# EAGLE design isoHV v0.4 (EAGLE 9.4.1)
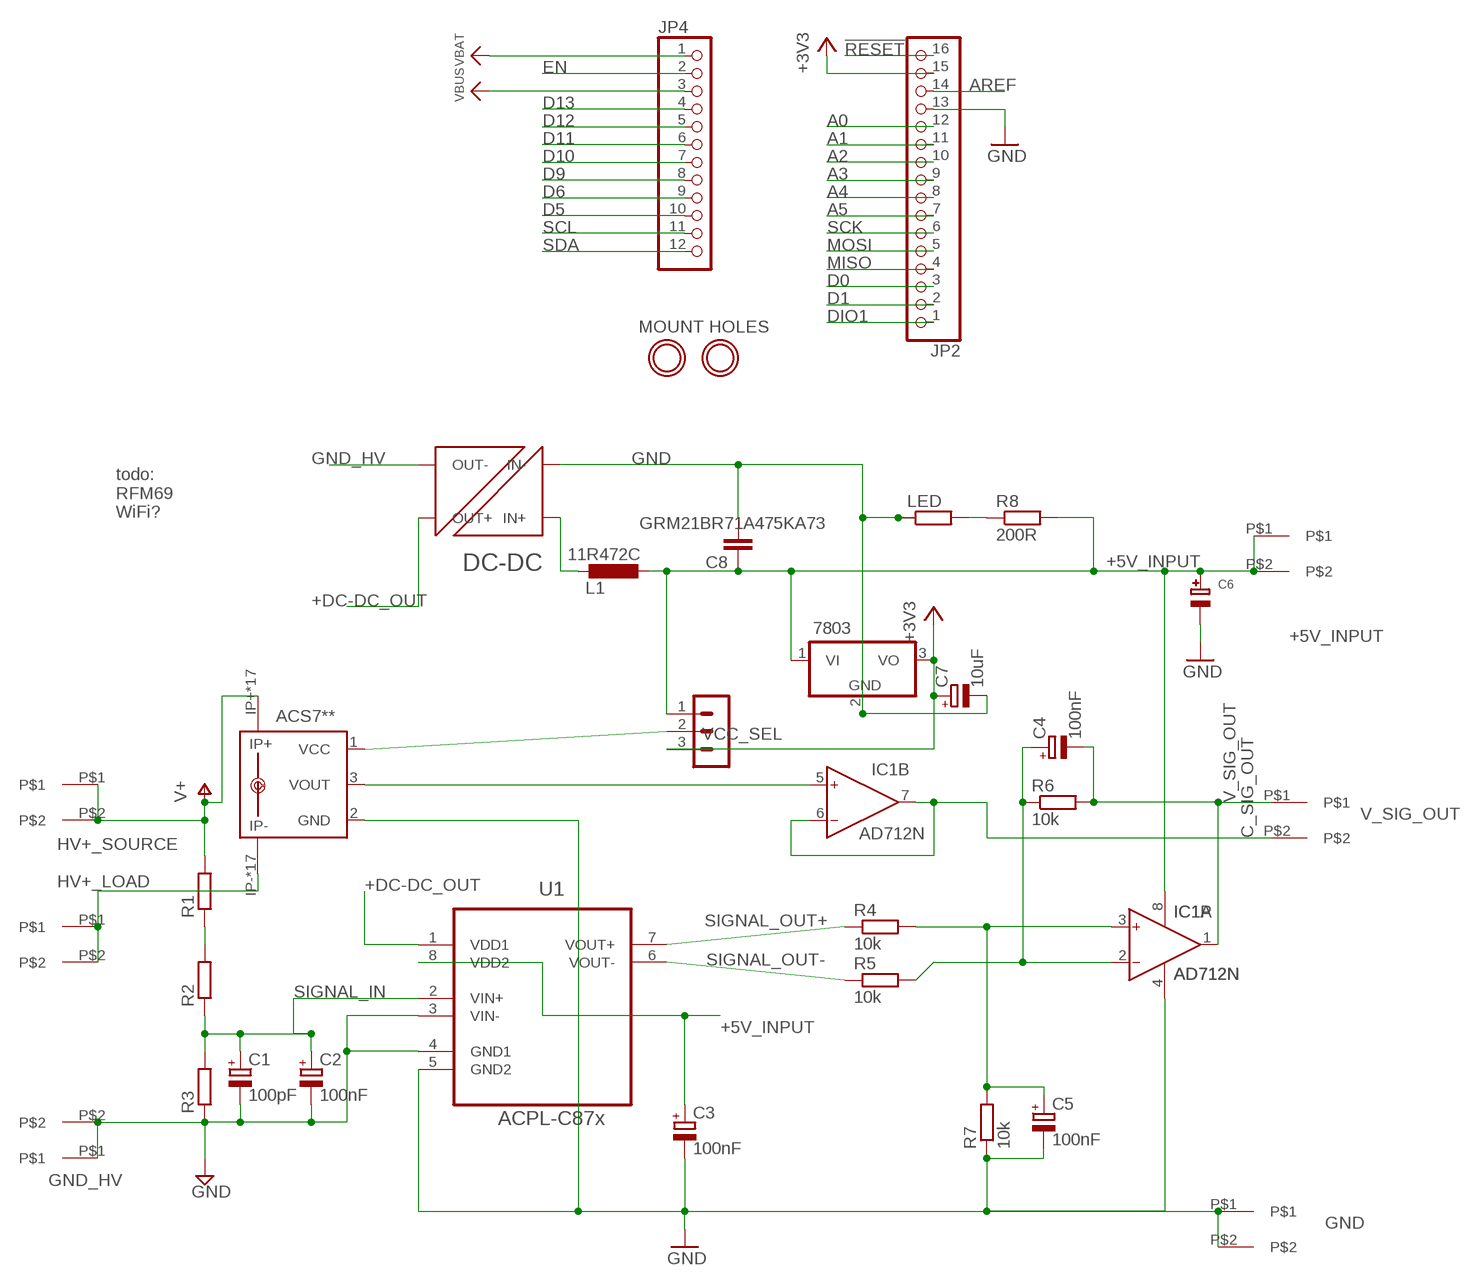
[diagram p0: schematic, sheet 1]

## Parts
7803  7805TV  [TO220V]
ACS7**  ACS758KCB-150B-PFF-T  [CB-PFF]
C1  100pF  CPOL-EUB45181A  [B45181A]
C2  100nF  CPOL-EUB45181A  [B45181A]
C3  100nF  CPOL-EUB45181A  [B45181A]
C4  100nF  CPOL-EUB45181A  [B45181A]
C5  100nF  CPOL-EUB45181A  [B45181A]
C6  CAP_ELECTROLYTICPTH_3.5MMGRID_10MMDIA  [CELEC_3.5MM_10MM]
C7  10uF  CPOL-EUB45181A  [B45181A]
C8  GRM21BR71A475KA73  C-EU025-050X050  [C025-050X050]
IC1  AD712N  [DIL08]
JP2  HEADER-1X16ROUND  [1X16_ROUND]
JP4  HEADER-1X12  [1X12_ROUND]
L1  11R472C  L-EU0204V  [0204V]
LED  R-EU_0204/2V  [0204V]
R1  R-EU_0411/15  [0411/15]
R2  R-EU_0411/15  [0411/15]
R3  R-EU_0411/15  [0411/15]
R4  10k  R-EU_0204/7  [0204/7]
R5  10k  R-EU_0204/7  [0204/7]
R6  10k  R-EU_0204/7  [0204/7]
R7  10k  R-EU_0204/7  [0204/7]
R8  200R  R-EU_0204/2V  [0204V]
U1  ACPL-C87x  ACPL-C79B-000E  [SOIC127P1150X330-8N]
U$1  7.62MM_TERMINAL_BLOCK  [7.62MM]
U$2  7.62MM_TERMINAL_BLOCK  [7.62MM]
U$3  7.62MM_TERMINAL_BLOCK  [7.62MM]
U$4  7.62MM_TERMINAL_BLOCK  [7.62MM]
U$5  7.62MM_TERMINAL_BLOCK  [7.62MM]
U$6  7.62MM_TERMINAL_BLOCK  [7.62MM]
U$7  NXF1  [NXF1]
U$12  MOUNTINGHOLE2.5  [MOUNTINGHOLE_2.5_PLATED]
U$13  MOUNTINGHOLE2.5  [MOUNTINGHOLE_2.5_PLATED]
VCC_SEL  MA03-1  [MA03-1]

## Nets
!RESET: JP2.16
+3V3: 7803.3(VO) C7.+ JP2.15 VCC_SEL.3
+5V_INPUT: 7803.1(VI) C3.+ C6.+ C8.1 IC1.8(P:V+) L1.2 R8.2 U1.8(VDD2) U$3.P$1 U$3.P$2 VCC_SEL.1
+DC-DC_OUT: U1.1(VDD1) U$7.P$8(OUT+)
A0: JP2.12
A1: JP2.11
A2: JP2.10
A3: JP2.9
A4: JP2.8
A5: JP2.7
AREF: JP2.14
C_SIG_OUT: IC1.6(B:IN-) IC1.7(B:OUT) U$5.P$2
D0: JP2.3
D1: JP2.2
D5: JP4.10
D6: JP4.9
D9: JP4.8
D10: JP4.7
D11: JP4.6
D12: JP4.5
D13: JP4.4
DIO1: JP2.1
EN: JP4.2
GND: 7803.2(GND) ACS7**.2(GND) C3.- C5.- C6.- C7.- C8.2 IC1.4(P:V-) JP2.13 LED.1 R7.1 U1.5(GND2) U$4.P$1 U$4.P$2 U$7.P$1(IN-)
GND_HV: C1.- C2.- R3.1 U1.3(VIN-) U1.4(GND1) U$2.P$1 U$2.P$2 U$7.P$7(OUT-) ; supply symbol labelled GND
HV+_LOAD: ACS7**.IP- ACS7**.IP-@2(IP-) ACS7**.IP-@3(IP-) ACS7**.IP-@4(IP-) ACS7**.IP-@5(IP-) ACS7**.IP-@6(IP-) ACS7**.IP-@7(IP-) ACS7**.IP-@8(IP-) ACS7**.IP-@9(IP-) ACS7**.IP-@10(IP-) ACS7**.IP-@11(IP-) ACS7**.IP-@12(IP-) ACS7**.IP-@13(IP-) ACS7**.IP-@14(IP-) ACS7**.IP-@15(IP-) ACS7**.IP-@16(IP-) ACS7**.IP-@17(IP-) U$6.P$1 U$6.P$2
HV+_SOURCE: ACS7**.IP+ ACS7**.IP+@2(IP+) ACS7**.IP+@3(IP+) ACS7**.IP+@4(IP+) ACS7**.IP+@5(IP+) ACS7**.IP+@6(IP+) ACS7**.IP+@7(IP+) ACS7**.IP+@8(IP+) ACS7**.IP+@9(IP+) ACS7**.IP+@10(IP+) ACS7**.IP+@11(IP+) ACS7**.IP+@12(IP+) ACS7**.IP+@13(IP+) ACS7**.IP+@14(IP+) ACS7**.IP+@15(IP+) ACS7**.IP+@16(IP+) ACS7**.IP+@17(IP+) R1.2 U$1.P$1 U$1.P$2 ; supply symbol labelled V+
MISO: JP2.4
MOSI: JP2.5
N$1: C5.+ IC1.3(A:IN+) R4.2 R7.2
N$2: R1.1 R2.2
N$3: ACS7**.1(VCC) VCC_SEL.2
N$4: LED.2 R8.1
N$5: C4.+ IC1.2(A:IN-) R5.2 R6.1
N$6: ACS7**.3(VOUT) IC1.5(B:IN+)
N$7: L1.1 U$7.P$3(IN+)
SCK: JP2.6
SCL: JP4.11
SDA: JP4.12
SIGNAL_IN: C1.+ C2.+ R2.1 R3.2 U1.2(VIN+)
SIGNAL_OUT+: R4.1 U1.7(VOUT+)
SIGNAL_OUT-: R5.1 U1.6(VOUT-)
V_SIG_OUT: C4.- IC1.1(A:OUT) R6.2 U$5.P$1
VBAT: JP4.1
VBUS: JP4.3

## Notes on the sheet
- MOUNT HOLES
- todo:
  RFM69
  WiFi?

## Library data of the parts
7803 = linear:78*: Positive VOLTAGE REGULATOR Source: http://cache.national.com/ds/LM/LM78L05.pdf http://www.fairchildsemi.com/ds/LM/LM7805.pdf
ACS7** = allegro:ACS758*: Thermally Enhanced, Fully Integrated, Hall Effect-Based Linear Current Sensor with 100 micro Ohm Current Conductor display layer 49 Reference in BRD and place VIAs on circles Source: http://www.allegromicro.com/en/Products/Part_Numbers/0758/0758.pdf; MPN: ACS7**; OC_FARNELL: 1718995; OC_NEWARK: 04R7129
C1-C5 C7 = rcl:CPOL-EU: POLARIZED CAPACITOR, European symbol; SPICEPREFIX: C
C6 = microbuilder:CAP_ELECTROLYTIC: Electrolytic Capacitors
C8 = rcl:C-EU: CAPACITOR, European symbol; SPICEPREFIX: C
IC1 = analog-devices:AD712: Dual Precision, Low Cost, High Speed BiFET Op Amp Source: http://www.analog.com/static/imported-files/data_sheets/AD712.pdf; MF: ALTERA CORPORATION; MPN: AD712JNZ; OC_FARNELL: 9604898; OC_NEWARK: 59K4554
JP2 = microbuilder:HEADER-1X16: PIN HEADER
JP4 = microbuilder:HEADER-1X12
L1 = rcl:L-EU: INDUCTOR, European symbol; SPICEPREFIX: L
LED R1-R8 = rcl:R-EU_: RESISTOR, European symbol; SPICEPREFIX: R
U1 = Avago_By_element14_Batch_1:ACPL-C79B-000E: Precision Miniature Isolation Amplifiers; DESCRIPTION: Precision Miniature Isolation Amplifiers; MPN: ACPL-C79B-000E; OC_FARNELL: 1854253; OC_NEWARK: 74R5803; PACKAGE: SOIC-8; SUPPLIER: AVAGO TECHNOLOGIES
U$1-U$6 = 7.62mm terminal block:7.62MM_TERMINAL_BLOCK
U$7 = NXF1:NXF1
U$12 U$13 = microbuilder:MOUNTINGHOLE: Mounting Hole
VCC_SEL = con-lstb:MA03-1: PIN HEADER; OC_FARNELL: unknown; OC_NEWARK: unknown

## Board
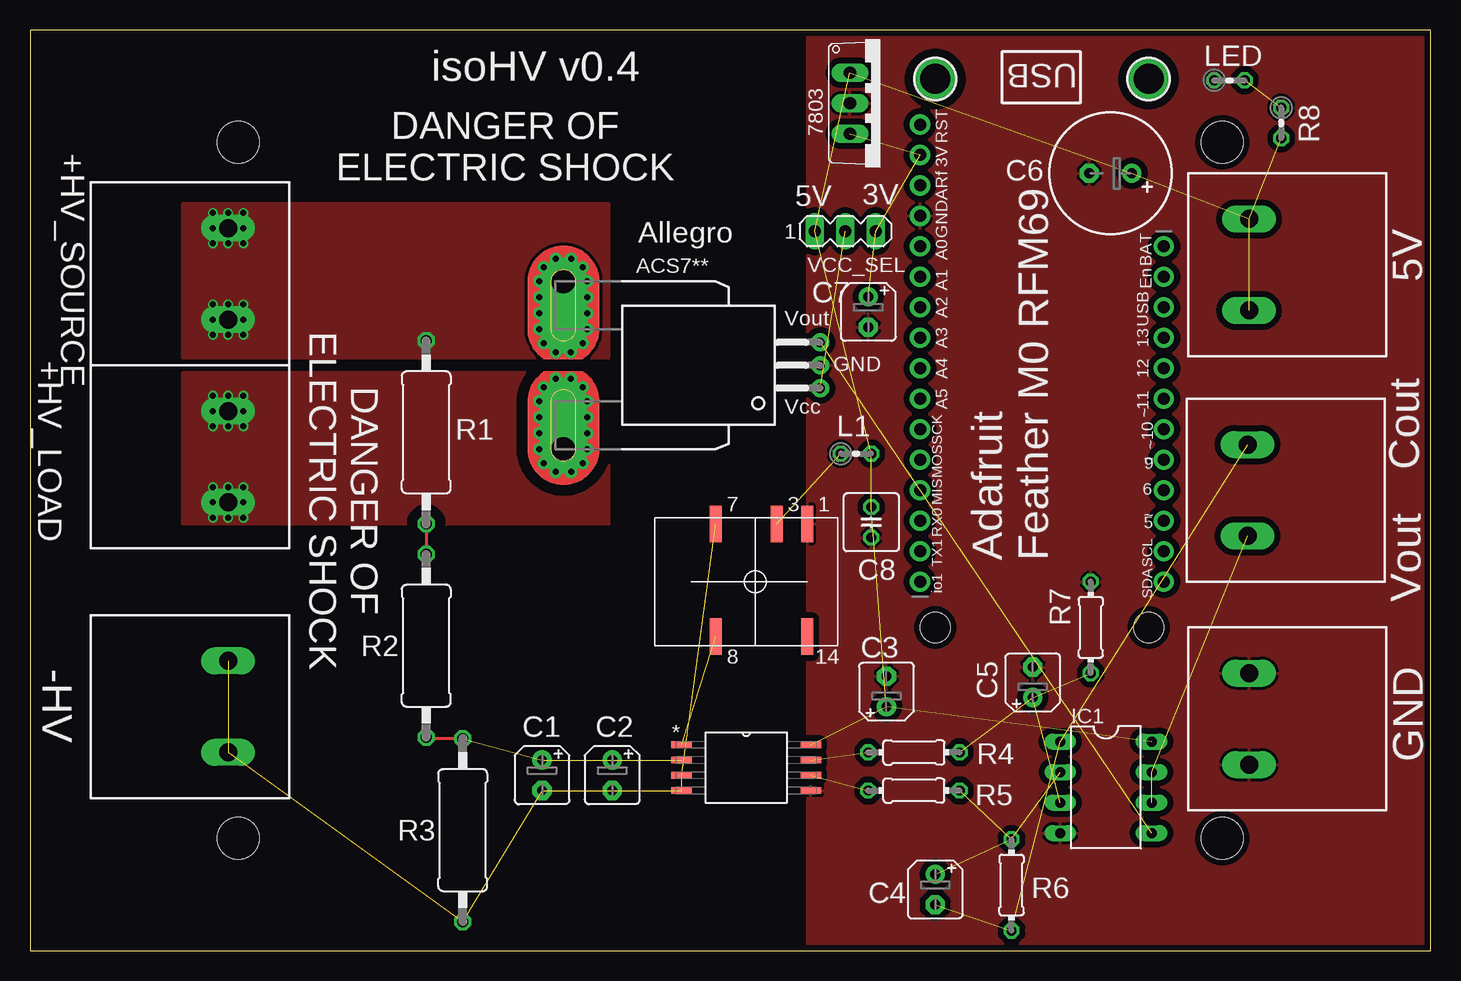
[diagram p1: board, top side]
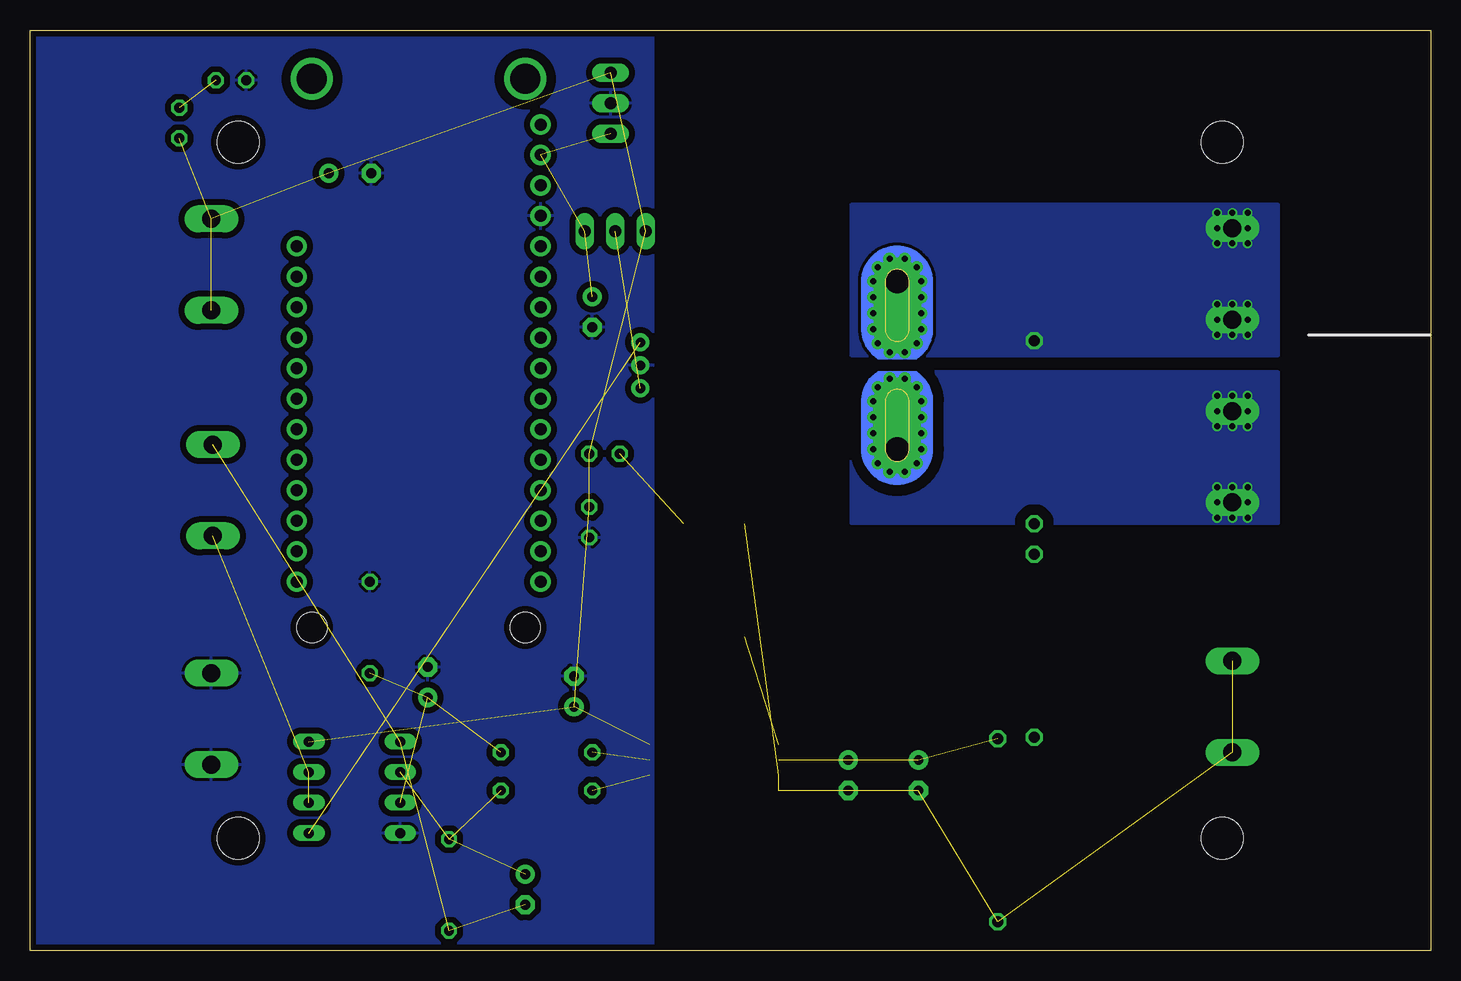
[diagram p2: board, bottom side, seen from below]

Size 116.71 x 76.71 mm. Coordinates in mm from the lower left corner, seen from the top.
Outline: 116.71,76.71 0,76.71 0,0 116.71,0 116.71,76.71
Copper layers (1*16): Top 0.07111875mm / dielectric 1.45776875mm / Bottom 0.07111875mm
Design rules "jlcpcb *": minimum track width 6mil, minimum drill 12mil, track to track 10mil, track to pad 10mil, pad to pad 10mil, via to via 10mil, smd to smd 0mil, copper to edge 10mil, drill to drill 10mil, minimum pad ring 10mil, minimum via ring 6mil, stop-mask expansion 2mil, vias tented up to drill 25mil, thermal gap 10mil
Holes 2.5 mm at 93.22,26.92 75.44,26.92
Holes 3.5 mm at 17.36,67.36 99.36,67.36 99.36,9.36 17.36,9.36

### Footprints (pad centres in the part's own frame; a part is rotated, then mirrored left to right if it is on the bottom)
TO220V = drill 1.016 long: 1 -2.54,-2.54; 2 0,-2.54; 3 2.54,-2.54
CB-PFF = drill 0.8 pad 1.5: 1 -1.91,-21.4; 2 0,-21.4; 3 1.91,-21.4 | drill 2 pad 4 offset: IP+ 7,0; IP- -7,0 | drill 0.5 pad 0.9: IP+@2 8.89,0.635; IP+@3 8.89,-0.635; IP+@4 8.175,-1.625; IP+@5 7,-2; IP+@6 5.675,-2; IP+@7 4.35,-2; IP+@8 3,-2; IP+@9 1.825,-1.625; IP+@10 1.1,-0.625; IP+@11 1.1,0.625; IP+@12 1.825,1.625; IP+@13 3,2; IP+@14 4.35,2; IP+@15 5.675,2; IP+@16 7,2; IP+@17 8.175,1.625; IP-@2 -8.89,0.635; IP-@3 -8.89,-0.635; IP-@4 -8.175,-1.625; IP-@5 -7,-2; IP-@6 -5.675,-2; IP-@7 -4.325,-2; IP-@8 -3,-2; IP-@9 -1.825,-1.625; IP-@10 -1.1,-0.625; IP-@11 -1.1,0.625; IP-@12 -1.825,1.625; IP-@13 -3,2; IP-@14 -4.325,2; IP-@15 -5.675,2; IP-@16 -7,2; IP-@17 -8.175,1.625
B45181A = drill 0.813 pad 1.6: + -1.27,0 | drill 0.813 pad 1.6 octagon: - 1.27,0
CELEC_3.5MM_10MM = drill 0.813 pad 1.6: + -1.778,0 | drill 0.813 pad 1.6 octagon: - 1.778,0
C025-050X050 = drill 0.813 octagon: 1 -1.27,0; 2 1.27,0
DIL08 = drill 0.813 long: 1 -3.81,-3.81; 2 -1.27,-3.81; 3 1.27,-3.81; 4 3.81,-3.81; 5 3.81,3.81; 6 1.27,3.81; 7 -1.27,3.81; 8 -3.81,3.81
1X16_ROUND = drill 1 pad 1.676: 1 -19.05,0; 2 -16.51,0; 3 -13.97,0; 4 -11.43,0; 5 -8.89,0; 6 -6.35,0; 7 -3.81,0; 8 -1.27,0; 9 1.27,0; 10 3.81,0; 11 6.35,0; 12 8.89,0; 13 11.43,0; 14 13.97,0; 15 16.51,0; 16 19.05,0
1X12_ROUND = drill 1 pad 1.676: 1 -13.97,0; 2 -11.43,0; 3 -8.89,0; 4 -6.35,0; 5 -3.81,0; 6 -1.27,0; 7 1.27,0; 8 3.81,0; 9 6.35,0; 10 8.89,0; 11 11.43,0; 12 13.97,0
0204V = drill 0.813 octagon: 1 -1.27,0; 2 1.27,0
0411/15 = drill 0.914 octagon: 1 -7.62,0; 2 7.62,0
0204/7 = drill 0.813 octagon: 1 -3.81,0; 2 3.81,0
SOIC127P1150X330-8N = smd 1.702 x 0.559: 1 -5.385,1.905; 2 -5.385,0.635; 3 -5.385,-0.635; 4 -5.385,-1.905; 5 5.385,-1.905; 6 5.385,-0.635; 7 5.385,0.635; 8 5.385,1.905
7.62MM = drill 1.5 long: P$1 0,-3.81; P$2 0,3.81
NXF1 = smd 0.991 x 3.048: P$1 0,0; P$3 2.54,0; P$7 7.62,0; P$8 7.62,9.398; P$14 0,9.398
MOUNTINGHOLE_2.5_PLATED = drill 2.5 pad 3.2: P$1 0,0
MA03-1 = drill 1.016 long: 1 -2.54,0; 2 0,0; 3 2.54,0

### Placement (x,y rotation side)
7803  70.87,70.61 270 top
ACS7**  44.45,48.77 90 top
C1  42.67,14.61 270 top
C2  48.51,14.61 270 top
C3  71.37,21.59 90 top
C4  75.44,5.08 270 top
C5  83.57,22.35 90 top
C6  90.04,64.77 180 top
C7  69.85,53.21 270 top
C8  70.1,35.69 270 top
IC1  89.66,13.59 270 top
JP2  74.17,49.78 90 top
JP4  94.49,44.7 270 top
L1  68.83,41.4 0 top
LED  99.95,72.52 0 top
R1  33.02,43.18 90 top
R2  33.02,25.4 90 top
R3  36.07,10.03 90 top
R4  73.66,16.51 0 top
R5  73.66,13.34 0 top
R6  81.79,5.46 270 top
R7  88.39,26.92 270 top
R8  104.27,68.96 270 top
U1  59.69,15.24 0 top
U$1  16.51,56.39 0 top
U$2  16.51,20.32 0 top
U$3  101.6,57.15 180 top
U$4  101.6,19.3 180 top
U$5  101.47,38.35 180 top
U$6  16.51,41.15 0 top
U$7  64.77,35.56 180 top
U$12  93.22,72.64 270 top
U$13  75.44,72.64 270 top
VCC_SEL  67.94,59.94 0 top

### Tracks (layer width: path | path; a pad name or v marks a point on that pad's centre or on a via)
+3V3  (3 unrouted)
+5V_INPUT  (10 unrouted)
+DC-DC_OUT  (1 unrouted)
C_SIG_OUT  (2 unrouted)
GND
  pour Bottom (isolate 0.508): 64.77,77.47 118.11,77.47 118.11,-1.27 64.77,-1.27
  pour Top (isolate 0.508): 64.77,78.74 64.77,-2.54 119.38,-2.54 119.38,78.74
GND_HV  (7 unrouted)
HV+_LOAD  (via drill 0.5)
  other vias: 16.51,43.69 15.24,46.23 16.51,46.23 17.78,46.23 17.78,44.96 17.78,43.69 15.24,43.69 15.24,44.96 17.78,38.61 17.78,37.34 17.78,36.07 16.51,36.07 15.24,36.07 15.24,37.34 15.24,38.61 16.51,38.61
  pour Bottom (isolate 0.889, no thermals): 48.26,48.26 12.7,48.26 12.7,35.56 48.26,35.56
  pour Top (isolate 0.889, no thermals): 48.26,48.13 12.7,48.13 12.7,35.56 48.26,35.56
HV+_SOURCE  (via drill 0.5)
  other vias: 15.24,53.85 16.51,53.85 17.78,53.85 17.78,52.58 17.78,51.31 16.51,51.31 15.24,51.31 15.24,52.58 16.51,58.93 17.78,58.93 17.78,60.2 17.78,61.47 16.51,61.47 15.24,61.47 15.24,60.2 15.24,58.93
  pour Bottom (no thermals): 12.7,49.53 48.26,49.53 48.26,62.23 12.7,62.23
  pour Top (no thermals): 12.7,49.4 48.26,49.4 48.26,62.23 12.7,62.23
N$1  (3 unrouted)
N$2
  Top 0.254: R1.1 R2.2
N$3  (1 unrouted)
N$4  (1 unrouted)
N$5  (3 unrouted)
N$6  (1 unrouted)
N$7  (1 unrouted)
SIGNAL_IN  (3 unrouted)
  Top 0.254: R2.1 33.15,17.65 R3.2
SIGNAL_OUT+  (1 unrouted)
SIGNAL_OUT-  (1 unrouted)
V_SIG_OUT  (3 unrouted)

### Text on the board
tPlace: USB | RST | 3V | ARf | GND | A0 | BAT | A1 | En | A2 | USB | A3 | 13 | A4 | 12 | A5 | 11 | ~ | SCK | 10 | ~ | MOS | 9 | ~ | MIS | 6 | RX0 | 5 | ~ | TX1 | Adafruit / Feather M0 RFM69 | SCL | io1 | SDA
tNames: isoHV v0.4 | DANGER OF / ELECTRIC SHOCK | +HV_SOURCE | 5V | 3V | Allegro | 5V | Vout | +HV_LOAD | GND | Vcc | Cout | DANGER OF / ELECTRIC SHOCK | Vout | -HV | GND

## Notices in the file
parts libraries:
microbuilder: This work is placed in the public domain, and may be freely used for commercial and non-commercial work with the following conditions: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
